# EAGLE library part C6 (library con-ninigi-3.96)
NINIGI
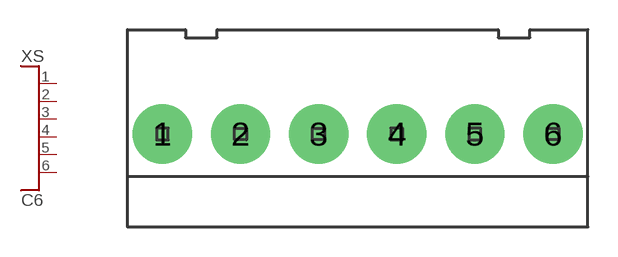
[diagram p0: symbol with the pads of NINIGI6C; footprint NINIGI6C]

Designator prefix XS

## C6  [NINIGI6C]
1  P$1
2  P$2
3  P$3
4  P$4
5  P$5
6  P$6

## Footprint NINIGI6C (pad centres in mm)
drill 1.6 pad 3: 1 -9.9,0; 2 -5.94,0; 3 -1.98,0; 4 1.98,0; 5 5.94,0; 6 9.9,0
